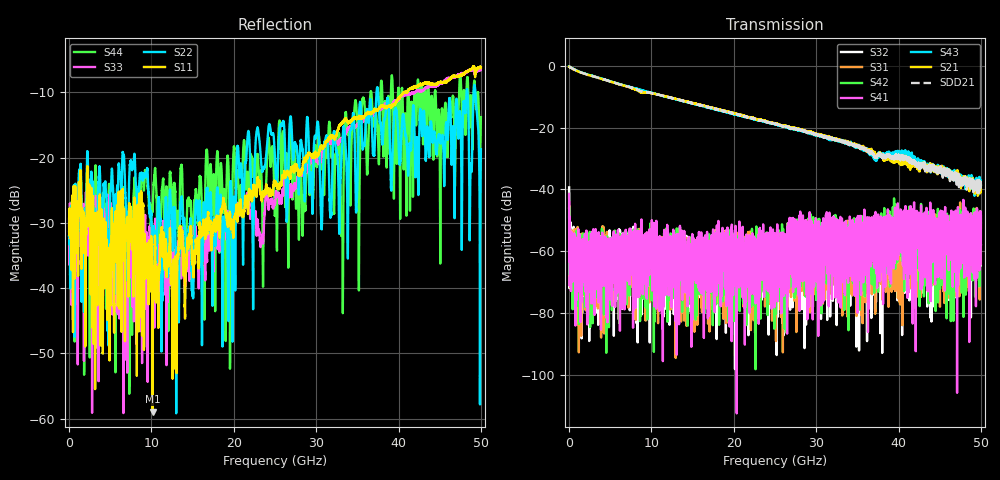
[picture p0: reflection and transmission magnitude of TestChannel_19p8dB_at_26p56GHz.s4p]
!Keysight Technologies,N5245A,MY49151038,A.10.65.06
!Date: Wednesday, June 07, 2023 11:15:15
!Correction: S11(Full 4 Port(1,2,3,4))
!S12(Full 4 Port(1,2,3,4))
!S13(Full 4 Port(1,2,3,4))
!S14(Full 4 Port(1,2,3,4))
!S21(Full 4 Port(1,2,3,4))
!S22(Full 4 Port(1,2,3,4))
!S23(Full 4 Port(1,2,3,4))
!S24(Full 4 Port(1,2,3,4))
!S31(Full 4 Port(1,2,3,4))
!S32(Full 4 Port(1,2,3,4))
!S33(Full 4 Port(1,2,3,4))
!S34(Full 4 Port(1,2,3,4))
!S41(Full 4 Port(1,2,3,4))
!S42(Full 4 Port(1,2,3,4))
!S43(Full 4 Port(1,2,3,4))
!S44(Full 4 Port(1,2,3,4))
!S4P File: Measurements: <S11,S12,S13,S14>,
!<S21,S22,S23,S24>,
!<S31,S32,S33,S34>,
!<S41,S42,S43,S44>:
# Hz S  RI  R 50
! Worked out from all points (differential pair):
!   5000 points, 10 MHz to 50 GHz, reference 50 ohm
!   strongest paths, dB at 10 MHz, 12.51 GHz, 25.01 GHz, 37.51 GHz, 50 GHz:
!     S21: -0.3, -10.4, -18.6, -28.6, -38.4
!     S43: -0.1, -10.4, -18.8, -29.3, -38.6
!     S41: -41.4, -61.9, -59.0, -54.7, -48.6
!     S42: -49.1, -75.5, -71.0, -58.0, -49.7
!     S31: -46.0, -65.7, -54.6, -64.0, -51.0
!     S32: -39.3, -57.4, -65.1, -69.7, -58.1
!   taken as a pair (ports 1,3 in; 2,4 out), SDD21 dB: -0.2, -10.4, -18.7, -28.9, -38.8
!   lowest |S11| = -58.9 dB at 10.15 GHz (marker M1), VSWR 1.00, Z = 50 + j0.109 ohm
!   |S11| at or under -10 dB: start of sweep to 40.7 GHz; 40.7137 GHz to 40.73245 GHz (18.76 MHz wide, 0.0461 % of centre); 40.86703 GHz to 40.91949 GHz (52.46 MHz wide, 0.128 % of centre)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
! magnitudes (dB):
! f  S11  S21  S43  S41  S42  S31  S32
! 10 MHz  -30.6  -0.3  -0.1  -41.4  -49.1  -46.0  -39.3
! 1.53 GHz  -34.0  -2.2  -2.2  -68.3  -60.7  -60.9  -88.2
! 7.47 GHz  -30.0  -7.1  -6.9  -60.2  -61.0  -61.4  -60.6
! 10.15 GHz  -58.9  -8.9  -8.8  -56.5  -57.7  -53.0  -56.9
! 37.45 GHz  -12.9  -29.2  -30.0  -61.3  -50.1  -58.7  -57.6
! 49.29 GHz  -7.6  -38.1  -40.2  -49.5  -55.2  -52.9  -56.4
! 50 GHz  -6.2  -38.4  -38.6  -48.6  -49.7  -51.0  -58.1
